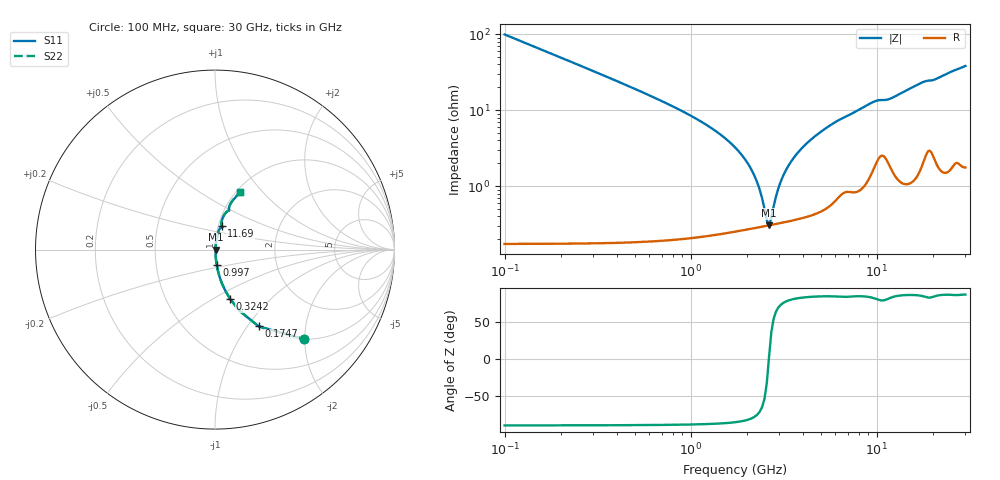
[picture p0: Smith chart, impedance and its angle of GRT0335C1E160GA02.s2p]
!Murata Part Number: GRT0335C1E160GA02
!These Parameters are Measured in Series Mode Connection
!Data Generated on Jun 19, 2026
!  o--ll--o
!Port1  Port2
!  o------o
!Operation Temp=25[degC], DC Bias Voltage=0[V]
!Freq. Start=100[MHz] Stop=30[GHz] 401[Steps]
# Hz S RI R 50
!Freq.(Hz) S11(Real) S11(Imag) S21(Real) S21(Imag) S12(Real) S12(Imag) S22(Real) S22(Imag)
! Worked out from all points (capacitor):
!   401 points, 100 MHz to 30 GHz, reference 50 ohm
!   read as one part in series: C = 16 pF near 249.5 MHz
!   lowest |Z| = 306 mohm at 2.642 GHz (marker M1)
!   series resonance near 2.635 GHz, so ESL is about 230 pH
!   S11 on the Smith chart (normalised r, x): 100 MHz: 1.00, -1.99; 174.8 MHz: 1.00, -1.13; 324.2 MHz: 1.00, -0.60; 997 MHz: 1.00, -0.17; 11.69 GHz: 1.04, +0.28; 30 GHz: 1.04, +0.76
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1e8  0.4966 -0.4991  0.5034 0.4991  0.5034 0.4991  0.4966 -0.4991
1.7475e8  0.2437 -0.4278  0.7563 0.4278  0.7563 0.4278  0.2437 -0.4278
3.2425e8  0.0849 -0.2759  0.9151 0.2759  0.9151 0.2759  0.0849 -0.2759
6.2325e8  0.0239 -0.1466  0.9761 0.1466  0.9761 0.1466  0.0239 -0.1466
9.97e8  0.00922 -0.0842  0.9908 0.0842  0.9908 0.0842  0.00922 -0.0842
1.96875e9  0.00314 -0.022  0.9969 0.022  0.9969 0.022  0.00314 -0.022
2.26775e9  0.00296 -0.0112  0.997 0.0112  0.997 0.0112  0.00296 -0.0112
2.492e9  0.00298 -0.00413  0.997 0.00413  0.997 0.00413  0.00298 -0.00413
2.6415e9  0.00304 0.000199  0.997 -0.000199  0.997 -0.000199  0.00304 0.000199
2.791e9  0.00314 0.00429  0.9969 -0.00429  0.9969 -0.00429  0.00314 0.00429
2.9405e9  0.00327 0.00817  0.9967 -0.00817  0.9967 -0.00817  0.00327 0.00817
3.09e9  0.00342 0.0119  0.9966 -0.0119  0.9966 -0.0119  0.00342 0.0119
3.46375e9  0.00391 0.0206  0.9961 -0.0206  0.9961 -0.0206  0.00391 0.0206
4.1365e9  0.00508 0.0346  0.9949 -0.0346  0.9949 -0.0346  0.00508 0.0346
5.10825e9  0.00753 0.0529  0.9925 -0.0529  0.9925 -0.0529  0.00753 0.0529
6.60325e9  0.014 0.0771  0.986 -0.0771  0.986 -0.0771  0.014 0.0771
1.01165e10  0.0375 0.125  0.9625 -0.125  0.9625 -0.125  0.0375 0.125
1.168625e10  0.0364 0.1314  0.9636 -0.1314  0.9636 -0.1314  0.0364 0.1314
1.505e10  0.045 0.181  0.955 -0.181  0.955 -0.181  0.045 0.181
2.005825e10  0.0783 0.2225  0.9217 -0.2225  0.9217 -0.2225  0.0783 0.2225
2.50665e10  0.1048 0.2813  0.8952 -0.2813  0.8952 -0.2813  0.1048 0.2813
3e10  0.1388 0.3234  0.8612 -0.3234  0.8612 -0.3234  0.1388 0.3234
